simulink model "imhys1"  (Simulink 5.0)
settings: Solver=ode45  StartTime=0.0  StopTime=1  MaxStep=2e-3  RelTol=1e-3
libraries: simulink x1

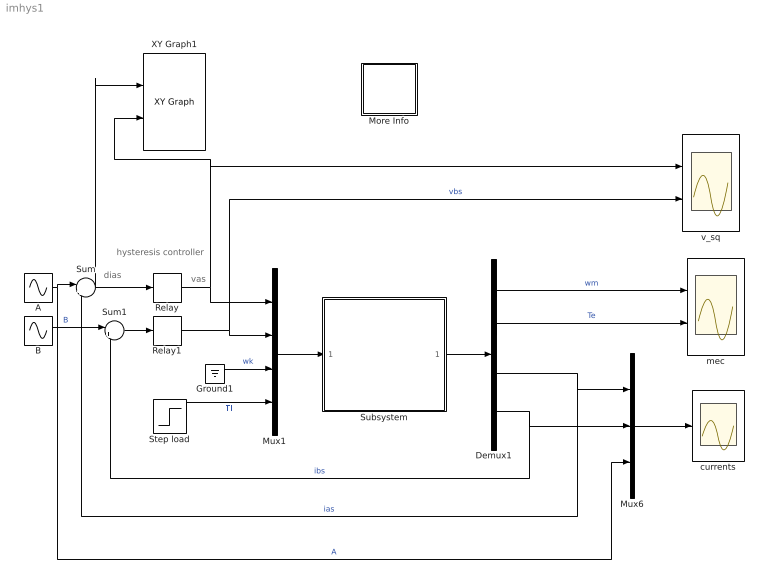
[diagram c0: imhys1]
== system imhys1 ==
  note: hysteresis controller
  note: vas
  note: dias
  A : Sin  Amplitude=1.5  Frequency=2*pi*50  Phase=pi/2  SampleTime=0
  B : Sin  Amplitude=1.5  Frequency=2*pi*50  SampleTime=0
  Demux1 : Demux
  Ground1 : Ground
  More Info : Subsystem
  Mux1 : Mux
  Mux6 : Mux  Inputs=3
  Relay : Relay  OnSwitchValue=0.1  OffSwitchValue=-0.1  OffOutputValue=-1
  Relay1 : Relay  OnSwitchValue=0.1  OffSwitchValue=-0.1  OffOutputValue=-1
  Step load : Step  Time=0.0  Before=0.0  After=0.25  SampleTime=0
  Subsystem : Subsystem  mask{Rs=0.01, Rr=0.02, L_param=[0.1 0.1 4.5], wo=2*pi*50, Hi=0.3, ic=[0.4517 -.0019 0.1778 0.004 0.98]}
      mask prompts: Rs "Stator resistance [pu]"; Rr "Rotor Resistance [pu]"; L_param "Inductances Lsl,Lrl,Lm[pu]"; wo "Base frequency [rad/s]"; Hi "Inertia Constant [s]"; ic "Initial Conditions"
  Sum : Sum  Inputs=|+-
  Sum1 : Sum  Inputs=|+-
  XY Graph1 : simulink/Sinks/XY Graph  xmin=-2  xmax=2  ymin=-1.5  ymax=1.5  st=0
  currents : Scope
  mec : Scope  NumInputPorts=2
  v_sq : Scope  NumInputPorts=2
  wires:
  Subsystem/1(Out1) -> Demux1/1
  Mux1/1 -> Subsystem/1(In1)
  Mux6/1 -> currents/1
  Demux1/1 -> mec/1  "wm"
  Demux1/2 -> mec/2  "Te"
  Demux1/3 -> Mux6/1, Sum/2  "ias"
  Ground1/1 -> Mux1/3  "wk"
  Step load/1 -> Mux1/4  "Tl"
  Relay1/1 -> Mux1/2, v_sq/2  "vbs"
  Relay/1 -> Mux1/1, v_sq/1, XY Graph1/2
  Sum1/1 -> Relay1/1
  B/1 -> Sum1/1  "B"
  Demux1/4 -> Mux6/2, Sum1/2  "ibs"
  Sum/1 -> Relay/1, XY Graph1/1
  A/1 -> Sum/1, Mux6/3  "A"

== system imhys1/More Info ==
  note: This demo simulates the characteristics of an induction motor under current controlled excitation

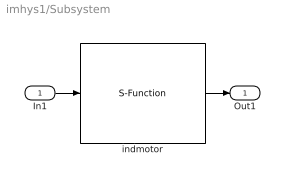
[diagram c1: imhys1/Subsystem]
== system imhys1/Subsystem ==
  In1 : Inport
  indmotor : S-Function  FunctionName=imKmod0  Parameters=Rs,Rr,L_param,Hi,wo,ic
  Out1 : Outport
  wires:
  indmotor/1 -> Out1/1
  In1/1 -> indmotor/1
